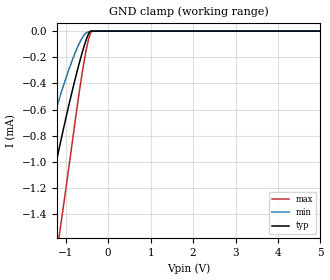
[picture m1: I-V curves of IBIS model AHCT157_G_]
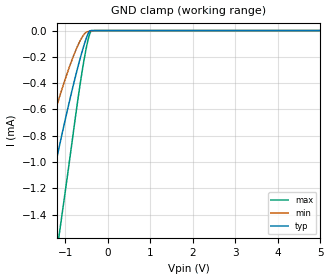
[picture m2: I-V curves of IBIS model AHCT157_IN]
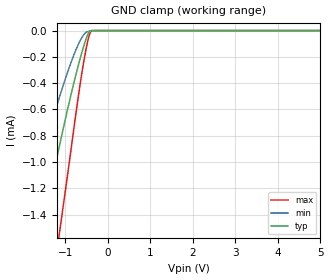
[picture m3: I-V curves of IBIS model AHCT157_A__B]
| TEXAS INSTRUMENTS INCORPORATED
| Standard Linear and Logic Group
| IBIS Model of SN74AHCT157
| QUADRUPLE 2-LINE TO 1-LINE DATA SELECTORS/MULTIPLEXERS
| This file contains package information for the following:
|  SOIC 16-pin (D) package as [Component] AHCT157_D
|  SSOP 16-pin (DB) package as [Component] AHCT157_DB
|  TVSOP 16-pin (DGV) package as [Component] AHCT157_DGV
|  PDIP 16-pin (N) package as [Component] AHCT157_N
|  TSSOP 16-pin (PW) package as [Component] AHCT157_PW
| This device can be powered at the following Vccs:
|  5 volt Vcc
| This file provides unique models under the [Model Selector] for each Vcc.
| For operation at a specific Vcc, select the appropriate model after each
| [Model Selector] keyword.
[IBIS Ver]   3.2
[Comment char]  |_char
[File Name]   sn74ahct157.ibs
[File Rev]   1.0 | a_die
[Date]   July 17, 2001
[Source]   Data created from TI-SPICE simulations at TI-SLL.
[Notes]   The following is an IBIS list for the AHCT157.
   Please contact sllibis@ti.com with questions and
   comments concerning SLL IBIS models.
   This IBIS model is created from a BA (back annotated netlist)
   -To comply with the data sheet we omitted the Vref
   and Rref from the Output Model
   -As there is no power clamp diode in the Input Model,
   we removed the Pwr Clamp table data from the Input Model
[Disclaimer] Property of Texas Instruments Incorporated.  Unauthorized
   reproduction and/or distribution is strictly prohibited.
   This product is protected under copyright law.
   Created  2001, (C) Copyright  2001, Texas Instruments
   Incorporated, All Rights Reserved
   UNLESS THERE IS A SIGNED, WRITTEN AGREEMENT TO THE
   CONTRARY, TEXAS INSTRUMENTS (TI) IS PROVIDING THE IBIS
   MODELS  AND WITHOUT ANY WARRANTY, EXPRESSED OR
   IMPLIED.  TI assumes no liability for:
   1) the accuracy of the IBIS models provided to your
   company;
   2) the proper functioning of these IBIS Models in your
   design or for any resulting applications; or
   3) infringement of patents, copyrights or intellectual
   property rights resulting from your use of these IBIS
   models.
   TI provides IBIS Models as a service to our customers.
   You and your company shall not distribute, sell or give
   these models to anyone else without prior written
   permission from TI.
   TI reserves the right to make changes to our products or
   to discontinue any semiconductor product or service
   without notice, and advises our customers to obtain the
   latest version of relevant information to verify, before
   placing orders, that the information being relied on is
   current.
   Please be aware that your receipt and use of the IBIS
   information provided shall serve as acceptance of these
   terms and conditions.  If you do not accept these terms,
   you should return or destroy the IBIS models and any
   other accompanying information immediately.
| Component AHCT157_D 16-pin SOIC
[Component]   AHCT157_D
[Manufacturer]   Texas Instruments, Inc.
[Package]
|   typ   min   max
R_pkg   3.900e-02   2.800e-02   4.900e-02
L_pkg   3.453e-09   2.350e-09   4.375e-09
C_pkg   5.210e-13   2.540e-13   7.080e-13
[Pin]   signal_name   model_name   R_pin   L_pin   C_pin
1   A_BAR_B   AHCT157_A__B   4.200e-02   4.336e-09   7.030e-13
2   1A   AHCT157_IN   4.900e-02   3.778e-09   6.340e-13
3   1B   AHCT157_IN   2.800e-02   3.449e-09   5.180e-13
4   1Y   AHCT157_OUT   2.900e-02   2.393e-09   2.540e-13
5   2A   AHCT157_IN   2.800e-02   2.350e-09   2.640e-13
6   2B   AHCT157_IN   4.800e-02   3.312e-09   4.830e-13
7   2Y   AHCT157_OUT   4.300e-02   3.629e-09   6.040e-13
8   GND   GND   4.400e-02   4.375e-09   7.080e-13
9   3Y   AHCT157_OUT   4.200e-02   4.336e-09   7.030e-13
10   3B   AHCT157_IN   4.900e-02   3.778e-09   6.340e-13
11   3A   AHCT157_IN   2.800e-02   3.449e-09   5.180e-13
12   4Y   AHCT157_OUT   2.900e-02   2.393e-09   2.550e-13
13   4B   AHCT157_IN   2.800e-02   2.350e-09   2.640e-13
14   4A   AHCT157_IN   4.800e-02   3.312e-09   4.830e-13
15   G_BAR   AHCT157_G_   4.300e-02   3.629e-09   6.040e-13
16   VCC   POWER   4.400e-02   4.375e-09   7.080e-13
| Component AHCT157_DB 16-pin SSOP
[Component]   AHCT157_DB
[Manufacturer]   Texas Instruments, Inc.
[Package]
|   typ   min   max
R_pkg   4.800e-02   4.600e-02   5.000e-02
L_pkg   3.536e-09   3.213e-09   3.798e-09
C_pkg   3.760e-13   3.140e-13   4.400e-13
[Pin]   signal_name   model_name   R_pin   L_pin   C_pin
1   A_BAR_B   AHCT157_A__B   4.800e-02   3.797e-09   3.770e-13
2   1A   AHCT157_IN   4.600e-02   3.723e-09   4.400e-13
3   1B   AHCT157_IN   4.800e-02   3.409e-09   3.720e-13
4   1Y   AHCT157_OUT   4.900e-02   3.213e-09   3.140e-13
5   2A   AHCT157_IN   4.900e-02   3.213e-09   3.140e-13
6   2B   AHCT157_IN   4.800e-02   3.409e-09   3.720e-13
7   2Y   AHCT157_OUT   4.600e-02   3.723e-09   4.400e-13
8   GND   GND   4.800e-02   3.798e-09   3.770e-13
9   3Y   AHCT157_OUT   4.800e-02   3.797e-09   3.770e-13
10   3B   AHCT157_IN   4.600e-02   3.725e-09   4.400e-13
11   3A   AHCT157_IN   4.800e-02   3.409e-09   3.720e-13
12   4Y   AHCT157_OUT   4.900e-02   3.214e-09   3.140e-13
13   4B   AHCT157_IN   5.000e-02   3.216e-09   3.140e-13
14   4A   AHCT157_IN   4.800e-02   3.409e-09   3.720e-13
15   G_BAR   AHCT157_G_   4.700e-02   3.729e-09   4.400e-13
16   VCC   POWER   4.800e-02   3.797e-09   3.770e-13
| Component AHCT157_DGV 16-pin TVSOP
[Component]   AHCT157_DGV
[Manufacturer]   Texas Instruments, Inc.
[Package]
|   typ   min   max
R_pkg   3.900e-02   3.300e-02   4.500e-02
L_pkg   2.543e-09   2.320e-09   2.938e-09
C_pkg   3.860e-13   3.340e-13   4.490e-13
[Pin]   signal_name   model_name   R_pin   L_pin   C_pin
1   A_BAR_B   AHCT157_A__B   3.500e-02   2.907e-09   4.170e-13
2   1A   AHCT157_IN   4.200e-02   2.558e-09   4.460e-13
3   1B   AHCT157_IN   3.800e-02   2.341e-09   3.450e-13
4   1Y   AHCT157_OUT   3.800e-02   2.320e-09   3.340e-13
5   2A   AHCT157_IN   3.900e-02   2.322e-09   3.340e-13
6   2B   AHCT157_IN   3.800e-02   2.353e-09   3.420e-13
7   2Y   AHCT157_OUT   4.000e-02   2.536e-09   4.410e-13
8   GND   GND   3.300e-02   2.897e-09   4.180e-13
9   3Y   AHCT157_OUT   3.500e-02   2.927e-09   4.190e-13
10   3B   AHCT157_IN   4.500e-02   2.632e-09   4.490e-13
11   3A   AHCT157_IN   3.900e-02   2.368e-09   3.470e-13
12   4Y   AHCT157_OUT   3.900e-02   2.330e-09   3.350e-13
13   4B   AHCT157_IN   3.900e-02   2.320e-09   3.350e-13
14   4A   AHCT157_IN   3.900e-02   2.361e-09   3.450e-13
15   G_BAR   AHCT157_G_   4.100e-02   2.573e-09   4.460e-13
16   VCC   POWER   3.500e-02   2.938e-09   4.200e-13
| Component AHCT157_N 16-pin PDIP
[Component]   AHCT157_N
[Manufacturer]   Texas Instruments, Inc.
[Package]
|   typ   min   max
R_pkg   5.600e-02   5.200e-02   6.300e-02
L_pkg   7.637e-09   5.451e-09   1.053e-08
C_pkg   5.280e-13   3.350e-13   8.930e-13
[Pin]   signal_name   model_name   R_pin   L_pin   C_pin
1   A_BAR_B   AHCT157_A__B   5.800e-02   1.053e-08   8.920e-13
2   1A   AHCT157_IN   6.200e-02   8.759e-09   5.350e-13
3   1B   AHCT157_IN   5.200e-02   7.146e-09   3.870e-13
4   1Y   AHCT157_OUT   5.300e-02   5.451e-09   4.080e-13
5   2A   AHCT157_IN   5.300e-02   5.513e-09   3.700e-13
6   2B   AHCT157_IN   5.300e-02   6.304e-09   3.360e-13
7   2Y   AHCT157_OUT   5.700e-02   7.830e-09   5.030e-13
8   GND   GND   5.600e-02   9.581e-09   8.050e-13
9   3Y   AHCT157_OUT   5.800e-02   9.603e-09   8.070e-13
10   3B   AHCT157_IN   6.200e-02   7.864e-09   5.030e-13
11   3A   AHCT157_IN   5.200e-02   6.295e-09   3.350e-13
12   4Y   AHCT157_OUT   5.300e-02   5.499e-09   3.560e-13
13   4B   AHCT157_IN   5.300e-02   5.452e-09   4.040e-13
14   4A   AHCT157_IN   5.300e-02   7.156e-09   3.870e-13
15   G_BAR   AHCT157_G_   6.300e-02   8.740e-09   5.340e-13
16   VCC   POWER   5.600e-02   1.048e-08   8.930e-13
| Component AHCT157_PW 16-pin TSSOP
[Component]   AHCT157_PW
[Manufacturer]   Texas Instruments, Inc.
[Package]
|   typ   min   max
R_pkg   4.500e-02   3.800e-02   5.100e-02
L_pkg   2.593e-09   2.447e-09   3.080e-09
C_pkg   2.810e-13   2.430e-13   3.770e-13
[Pin]   signal_name   model_name   R_pin   L_pin   C_pin
1   A_BAR_B   AHCT157_A__B   4.000e-02   3.080e-09   3.770e-13
2   1A   AHCT157_IN   3.800e-02   2.458e-09   2.810e-13
3   1B   AHCT157_IN   5.100e-02   2.512e-09   2.550e-13
4   1Y   AHCT157_OUT   5.100e-02   2.447e-09   2.430e-13
5   2A   AHCT157_IN   5.100e-02   2.447e-09   2.430e-13
6   2B   AHCT157_IN   5.100e-02   2.512e-09   2.550e-13
7   2Y   AHCT157_OUT   3.800e-02   2.458e-09   2.810e-13
8   GND   GND   4.000e-02   3.080e-09   3.770e-13
9   3Y   AHCT157_OUT   3.900e-02   2.832e-09   3.160e-13
10   3B   AHCT157_IN   3.800e-02   2.460e-09   2.790e-13
11   3A   AHCT157_IN   5.100e-02   2.512e-09   2.550e-13
12   4Y   AHCT157_OUT   5.100e-02   2.447e-09   2.430e-13
13   4B   AHCT157_IN   5.100e-02   2.447e-09   2.430e-13
14   4A   AHCT157_IN   5.100e-02   2.512e-09   2.550e-13
15   G_BAR   AHCT157_G_   3.800e-02   2.459e-09   2.790e-13
16   VCC   POWER   3.900e-02   2.832e-09   3.160e-13
| Models and submodels in the file (4): AHCT157_G_ (Input), AHCT157_IN (Input), AHCT157_A__B (Input), AHCT157_OUT (Output)
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[Model]   AHCT157_G_
Model_type  Input
Vinl = 0.8
Vinh = 2.0
| variable   typ   min   max
C_comp   0.74pF   0.55pF   0.86pF
[Temperature Range]   40   100   -40
| Ambient temperature   25   85   -40
[Voltage range]   5   4.5   5.5
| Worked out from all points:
|   GND clamp passes 1 mA (typ) near -1.22 V on its own axis
[GND Clamp]
| AHCT157_G_
|   Voltage   I(typ)   I(min)   I(max)
-5V       -7.629mA   -5.516mA   -11.13mA
-2.015V   -2.282mA   -1.522mA   -3.594mA
-1.595V   -1.587mA   -1.014mA   -2.593mA
-1.535V   -1.491mA   -943.8uA   -2.453mA
-1.15V    -892uA     -517.1uA   -1.562mA
-1.1V     -817.8uA   -465.4uA   -1.447mA
-760mV    -345uA     -153uA     -648.8uA
-615mV    -169.1uA   -54.76uA   -327.9uA
-495mV    -46.99uA   -9.753uA   -110.7uA
-430mV    -4.75uA    -5.225uA   -28.25uA
-380mV    -49.72nA   -2.663uA   -32.67nA
5V        14.12pA    103.7pA    10pA
[Model]   AHCT157_IN
Model_type  Input
Vinl = 0.8
Vinh = 2.0
| variable   typ   min   max
C_comp   0.69pF   0.51pF   0.79pF
[Temperature Range]   40   100   -40
| Ambient temperature   25   85   -40
[Voltage range]   5   4.5   5.5
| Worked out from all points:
|   GND clamp passes 1 mA (typ) near -1.22 V on its own axis
[GND Clamp]
| AHCT157_IN
|   Voltage   I(typ)   I(min)   I(max)
-5V       -7.629mA   -5.516mA   -11.13mA
-2.015V   -2.282mA   -1.522mA   -3.594mA
-1.595V   -1.587mA   -1.014mA   -2.593mA
-1.535V   -1.491mA   -943.8uA   -2.453mA
-1.15V    -892uA     -517.1uA   -1.562mA
-1.1V     -817.8uA   -465.4uA   -1.447mA
-760mV    -345uA     -153uA     -648.8uA
-615mV    -169.1uA   -54.76uA   -327.9uA
-495mV    -46.99uA   -9.753uA   -110.7uA
-430mV    -4.75uA    -5.225uA   -28.25uA
-380mV    -49.72nA   -2.663uA   -32.67nA
5V        14.12pA    103.7pA    10pA
[Model]   AHCT157_A__B
Model_type  Input
Vinl = 0.8
Vinh = 2.0
| variable   typ   min   max
C_comp   0.71pF   0.53pF   0.82pF
[Temperature Range]   40   100   -40
| Ambient temperature   25   85   -40
[Voltage range]   5   4.5   5.5
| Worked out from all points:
|   GND clamp passes 1 mA (typ) near -1.22 V on its own axis
[GND Clamp]
| AHCT157_A__B
|   Voltage   I(typ)   I(min)   I(max)
-5V       -7.629mA   -5.516mA   -11.13mA
-2.015V   -2.282mA   -1.522mA   -3.594mA
-1.595V   -1.587mA   -1.014mA   -2.593mA
-1.535V   -1.491mA   -943.8uA   -2.453mA
-1.15V    -892uA     -517.1uA   -1.562mA
-1.1V     -817.8uA   -465.4uA   -1.447mA
-760mV    -345uA     -153uA     -648.8uA
-615mV    -169.1uA   -54.76uA   -327.9uA
-495mV    -46.99uA   -9.753uA   -110.7uA
-430mV    -4.75uA    -5.225uA   -28.25uA
-380mV    -49.72nA   -2.663uA   -32.67nA
5V        14.12pA    103.7pA    10pA
